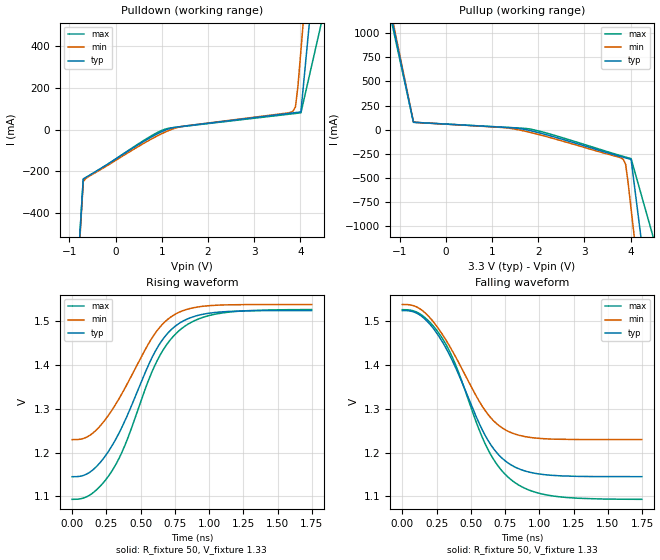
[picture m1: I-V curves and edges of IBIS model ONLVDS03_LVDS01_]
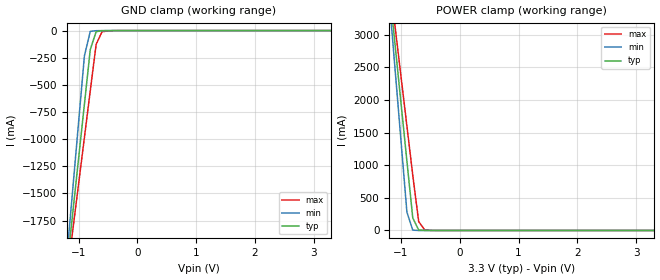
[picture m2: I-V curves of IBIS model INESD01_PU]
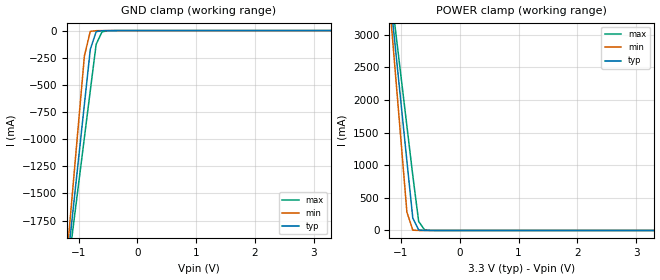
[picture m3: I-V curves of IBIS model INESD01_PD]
|   This file is an IBIS representation of the   |
|   Integrated Device Technology, Inc.   |
|   ICS844008I-01   |
|   FEMTOCLOCKS CRYSTAL-TO-LVDS FREQUENCY SYNTHESIZER   |
[IBIS Ver]   4.1
[File name]   844008i_01_3v3.ibs
[File Rev]   4.0
[Date]   15 Jul 2009 | Last modified
|   Mar 27 2006 | Generated
[Source]   Originated at Integrated Device Technology, Inc.
[Disclaimer]
IDT hereby grants the user of this IBIS model a non-exclusive,
nontransferable license to use this IBIS model under the following terms.
Before using this IBIS model, the user should read this license.
If the user does not accept these terms,  the IBIS model should be
returned to IDT within 30 days.
   The user is granted this license only to use the IBIS model and
is not granted rights to sell, load, rent, lease or license the IBIS
model in whole or in part, or in modified form to anyone other than
user. User may modify the IBIS model to suit its specific
applications but rights to derivative works and such modifications
shall belong to IDT.
   This IBIS model is provided on an "AS IS" basis and IDT makes
absolutely no warranty with respect to the information contained
herein. IDT DISCLAIMS AND CUSTOMER WAIVES ALL WARRANTIES, EXPRESS
OR IMPLIED, INCLUDING WARRANTIES OF MERCHANTABILITY OR FITNESS FOR
A PARTICULAR PURPOSE. The entire risk as to quality and performance
is with the Customer. ACCORDINGLY, IN NO EVENT SHALL THE COMPANY BE
LIABLE FOR ANY DAMAGES, WHETHER IN CONTRACT OR TORT,INCLUDING ANY
LOST PROFITS OR OTHER INCIDENTAL, CONSEQUENTIAL, EXEMPLARY, OR
PUNITIVE DAMAGES ARISING OUT OF THE USE OR APPLICATION OF THE IBIS
model provided in this package. Further, IDT reserves the right to
make changes without notice to any product herein to improve
reliability, function, or design. IDT does not convey any license
under patent rights or any other intellectual property rights,
including those of third parties.
   IDT is not obligated to provide maintenance or support
for the licensed IBIS model.
[Copyright]   Copyright 2008 by Integrated Device Technology, Inc.
[Component]   ICS844008YI-01
[Manufacturer] Integrated Device Technology, Inc.
[Package]
|LQFP32
|lead + wire   typ   min   max
R_pkg   220.4m   212.5m   238m
L_pkg   1.841n   1.708n   1.974n
C_pkg   0.316p   0.2907p   0.33p
[Pin] signal_name   model_name   R_pin   L_pin   C_pin
1   QA0   ONLVDS03_LVDS01_   238m   1.974n   0.330p
2   nQA0   ONLVDS03_LVDS01_   225m   1.841n   0.311p
3   VDD   POWER   218m   1.7745n   0.301p
4   QA1   ONLVDS03_LVDS01_   213m   1.708n   0.291p
5   nQA1   ONLVDS03_LVDS01_   213m   1.708n   0.291p
6   GND   GND   218m   1.7745n   0.301p
7   QA2   ONLVDS03_LVDS01_   225m   1.841n   0.311p
8   nQA2   ONLVDS03_LVDS01_   238m   1.974n   0.330p
9   F_SEL   INESD01_PU   238m   1.974n   0.330p
10   QA3   ONLVDS03_LVDS01_   225m   1.841n   0.311p
11   nQA3   ONLVDS03_LVDS01_   218m   1.7745n   0.301p
12   VDD   POWER   213m   1.708n   0.291p
13   GND   GND   213m   1.708n   0.291p
14   QB0   ONLVDS03_LVDS01_   218m   1.7745n   0.301p
15   nQB0   ONLVDS03_LVDS01_   225m   1.841n   0.311p
16   MR   INESD01_PD   238m   1.974n   0.330p
17   nQB1   ONLVDS03_LVDS01_   238m   1.974n   0.330p
18   QB1   ONLVDS03_LVDS01_   225m   1.841n   0.311p
19   GND   GND   218m   1.7745n   0.301p
20   nQB2   ONLVDS03_LVDS01_   213m   1.708n   0.291p
21   QB2   ONLVDS03_LVDS01_   213m   1.708n   0.291p
22   VDD   POWER   218m   1.7745n   0.301p
23   nQB3   ONLVDS03_LVDS01_   225m   1.841n   0.311p
24   QB3   ONLVDS03_LVDS01_   238m   1.974n   0.330p
25   VDDA   POWER   238m   1.974n   0.330p
26   nPLL_SEL   INESD01_PD   225m   1.841n   0.311p
27   VDD   POWER   218m   1.7745n   0.301p
28   OEB   INESD01_PU   213m   1.708n   0.291p
29   GND   GND   213m   1.708n   0.291p
30   XTAL_OUT   nc   218m   1.7745n   0.301p
31   XTAL_IN   nc   225m   1.841n   0.311p
32   OEA   INESD01_PU   238m   1.974n   0.330p
[Diff Pin]  inv_pin  vdiff tdelay_typ tdelay_min  tdelay_max
|Outputs
1   2   NA   0  0  0
4   5   NA   0  0  0
7   8   NA   0  0  0
10   11   NA   0  0  0
14   15   NA   0  0  0
18   17   NA   0  0  0
21   20   NA   0  0  0
24   23   NA   0  0  0
[Component]   ICS844008KI-01
[Manufacturer] Integrated Device Technology, Inc.
[Package]
|LD QFN 32
|lead + wire   typ   min   max
R_pkg   72.4655m   58.886m   86.045m
L_pkg   1.47175nH   1.11650nH   1.77850nH
C_pkg   0.07747pF   0.07444pF   0.08050pF
[Pin] signal_name   model_name   R_pin   L_pin   C_pin
1   QA0   ONLVDS03_LVDS01_   86.045m   1.77850nH   0.08050pF
2   nQA0   ONLVDS03_LVDS01_   76.996m   1.55783nH   0.07848pF
3   VDD   POWER   67.941m   1.33717nH   0.07646pF
4   QA1   ONLVDS03_LVDS01_   58.886m   1.11650nH   0.07444pF
5   nQA1   ONLVDS03_LVDS01_   58.886m   1.11650nH   0.07444pF
6   GND   GND   67.941m   1.33717nH   0.07646pF
7   QA2   ONLVDS03_LVDS01_   76.996m   1.55783nH   0.07848pF
8   nQA2   ONLVDS03_LVDS01_   86.045m   1.77850nH   0.08050pF
9   F_SEL   INESD01_PU   86.045m   1.77850nH   0.08050pF
10   QA3   ONLVDS03_LVDS01_   76.996m   1.55783nH   0.07848pF
11   nQA3   ONLVDS03_LVDS01_   67.941m   1.33717nH   0.07646pF
12   VDD   POWER   58.886m   1.11650nH   0.07444pF
13   GND   GND   58.886m   1.11650nH   0.07444pF
14   QB0   ONLVDS03_LVDS01_   67.941m   1.33717nH   0.07646pF
15   nQB0   ONLVDS03_LVDS01_   76.996m   1.55783nH   0.07848pF
16   MR   INESD01_PD   86.045m   1.77850nH   0.08050pF
17   nQB1   ONLVDS03_LVDS01_   86.045m   1.77850nH   0.08050pF
18   QB1   ONLVDS03_LVDS01_   76.996m   1.55783nH   0.07848pF
19   GND   GND   67.941m   1.33717nH   0.07646pF
20   nQB2   ONLVDS03_LVDS01_   58.886m   1.11650nH   0.07444pF
21   QB2   ONLVDS03_LVDS01_   58.886m   1.11650nH   0.07444pF
22   VDD   POWER   67.941m   1.33717nH   0.07646pF
23   nQB3   ONLVDS03_LVDS01_   76.996m   1.55783nH   0.07848pF
24   QB3   ONLVDS03_LVDS01_   86.045m   1.77850nH   0.08050pF
25   VDDA   POWER   86.045m   1.77850nH   0.08050pF
26   nPLL_SEL   INESD01_PD   76.996m   1.55783nH   0.07848pF
27   VDD   POWER   67.941m   1.33717nH   0.07646pF
28   OEB   INESD01_PU   58.886m   1.11650nH   0.07444pF
29   GND   GND   58.886m   1.11650nH   0.07444pF
30   XTAL_OUT   nc   67.941m   1.33717nH   0.07646pF
31   XTAL_IN   nc   76.996m   1.55783nH   0.07848pF
32   OEA   INESD01_PU   86.045m   1.77850nH   0.08050pF
[Diff Pin]  inv_pin  vdiff tdelay_typ tdelay_min  tdelay_max
|Outputs
1   2   NA   0  0  0
4   5   NA   0  0  0
7   8   NA   0  0  0
10   11   NA   0  0  0
14   15   NA   0  0  0
18   17   NA   0  0  0
21   20   NA   0  0  0
24   23   NA   0  0  0
| Models and submodels in the file (3): ONLVDS03_LVDS01_ (Output), INESD01_PU (Input), INESD01_PD (Input)
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[Model]   ONLVDS03_LVDS01_
Model_type   Output
Polarity   Non-Inverting
|   typ   min   max
C_comp   2pF   1.5pF   2.5pF
Vmeas = 1.33V
Rref = 50
Cref = 0
Vref = 1.33V
|   typ   min   max
[Voltage range]   3.3V   3.135V   3.465V
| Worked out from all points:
|   slope of the pulldown table from 0 to 0.495 V, typ, clamps not added: 7.11 ohm
|   slope of the pullup table from 0 to 0.495 V, typ, clamps not added: 37.1 ohm
|   rising waveform, R_fixture 50, V_fixture 1.33: 20-80 % time 339ps typ, 337ps min, 345ps max; typ from 1.15 V to 1.52 V
|   falling waveform, R_fixture 50, V_fixture 1.33: 20-80 % time 339ps typ, 337ps min, 345ps max; typ from 1.52 V to 1.15 V
[Pulldown]
|Voltage   I (typ)   I (min)   I (max)
-3.3V     -12.67A    -10.97A    -15.57A
-1.22V    -2.155A    -2.213A    -2.102A
-700mV    -236.2mA   -248.3mA   -238.7mA
-591mV    -221.6mA   -225.9mA   -223.9mA
921.3mV   -17.61mA   -27.52mA   -11.29mA
1.407V    15.22mA    14.4mA     14.35mA
3.838V    80.8mA     88.77mA    76.77mA
3.892V    82.3mA     109.8mA    78.15mA
3.946V    83.87mA    209.4mA    79.54mA
4.01V     86.01mA    380.6mA    81.18mA
4.528V    1.295A     1.771A     585.9mA
6.6V      7.985A     7.361A     9.102A
[Pullup]
|Voltage   I (typ)   I (min)   I (max)
-3.3V     7.977A     6.909A     9.772A
-1.22V    1.262A     1.3A       1.22A
-700mV    78.05mA    82.13mA    76.54mA
1.245V    25.16mA    22.28mA    26.55mA
1.786V    -4.761mA   -23mA      9.927mA
3.784V    -277.4mA   -290.3mA   -268.2mA
3.838V    -284.5mA   -305.2mA   -275.7mA
3.892V    -291.6mA   -357.9mA   -283.1mA
3.946V    -298.7mA   -552mA     -290.5mA
4.01V     -307.4mA   -820.6mA   -299.1mA
4.528V    -2.265A    -2.995A    -1.179A
6.6V      -12.7A     -11.71A    -14.49A
[Ramp]
|   typ   min   max
dV/dt_r   0.303/0.524n   0.247/0.507n   0.346/0.557n
dV/dt_f   0.303/0.524n   0.247/0.507n   0.346/0.557n
R_load =   50.0000
[Rising Waveform]
R_fixture = 50
V_fixture = 1.33   |Vcc_typ
V_fixture_min = 1.36 |Vcc_min
V_fixture_max = 1.33 |Vcc_max
C_fixture = 0.0p
| Time   typ   min   max
0s        1.145V     1.229V     1.093V
141.9ps   1.158V     1.242V     1.106V
289ps     1.214V     1.296V     1.157V
388.9ps   1.275V     1.349V     1.219V
613.1ps   1.435V     1.476V     1.405V
700.7ps   1.474V     1.505V     1.451V
798.8ps   1.498V     1.523V     1.483V
924.9ps   1.514V     1.533V     1.506V
1.093ns   1.521V     1.537V     1.519V
1.748ns   1.524V     1.538V     1.527V
[Falling Waveform]
R_fixture = 50
V_fixture = 1.33   |Vcc_typ
V_fixture_min = 1.36 |Vcc_min
V_fixture_max = 1.33 |Vcc_max
C_fixture = 0.0p
| Time   typ   min   max
0s        1.525V     1.539V     1.527V
141.9ps   1.512V     1.526V     1.515V
289ps     1.455V     1.472V     1.463V
388.9ps   1.395V     1.419V     1.401V
613.1ps   1.235V     1.293V     1.215V
700.7ps   1.196V     1.263V     1.169V
798.8ps   1.171V     1.245V     1.137V
924.9ps   1.156V     1.235V     1.115V
1.093ns   1.148V     1.231V     1.101V
1.748ns   1.145V     1.23V      1.093V
[Model]   INESD01_PU
Model_type   Input
Polarity   Non-Inverting
Vinl = 0.8V
Vinh = 2.0V
|   typ   min   max
C_comp   2pF   1.5pF   2.5pF
|   typ   min   max
[Voltage range]  3.3V   3.15V   3.45V
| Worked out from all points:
|   GND clamp passes 1 mA (typ) near -0.55 V on its own axis
|   POWER clamp passes 1 mA (typ) near -0.61 V on its own axis
[GND_clamp]
|Voltage   I(typ)   I(min)   I(max)
-3.3V     -12.83A    -15.14A    -11.37A
-1.2V     -2.195A    -2.092A    -2.281A
-1.1V     -1.689A    -1.472A    -1.849A
-900mV    -678.5mA   -232.7mA   -984.8mA
-800mV    -174mA     -7.237mA   -553.3mA
-700mV    -9.767mA   -1.114mA   -126.1mA
-600mV    -1.7mA     -240.1uA   -11.15mA
-300mV    -81.66uA   -67.79uA   -163.4uA
3.3V      1.866nA    1.113pA    239.1nA
[POWER_clamp]
|Voltage   I(typ)   I(min)   I(max)
-3.3V     22.38A     26.45A     19.82A
-1.2V     3.723A     3.545A     3.874A
-1.1V     2.836A     2.457A     3.116A
-1V       1.949A     1.369A     2.358A
-900mV    1.063A     281mA      1.601A
-800mV    191.5mA    5.012mA    843.9mA
-700mV    8.032mA    142.2uA    138.3mA
-600mV    607uA      17.63uA    10.62mA
-400mV    16.32uA    7.545uA    335.9uA
3.3V      -71.13uA   -62.11uA   -78.26uA
[Model]   INESD01_PD
Model_type   Input
Polarity   Non-Inverting
Vinl = 0.80V
Vinh = 2.0V
|   typ   min   max
C_comp   2pF   1.5pF   2.5pF
|   typ   min   max
[Voltage range]  3.3V   3.15V   3.45V
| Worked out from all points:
|   GND clamp passes 1 mA (typ) near -0.55 V on its own axis
|   POWER clamp passes 1 mA (typ) near -0.60 V on its own axis
[GND_clamp]
|Voltage I(typ)   I(min)   I(max)
-3.3V     -12.83A    -15.14A    -11.37A
-1.2V     -2.195A    -2.092A    -2.281A
-1.1V     -1.689A    -1.472A    -1.849A
-900mV    -678.5mA   -232.6mA   -984.8mA
-800mV    -173.9mA   -7.175mA   -553.2mA
-700mV    -9.696mA   -1.052mA   -126mA
-600mV    -1.629mA   -178uA     -11.07mA
-300mV    -10.53uA   -5.678uA   -86.08uA
3.3V      71.13uA    62.11uA    77.58uA
[POWER_clamp]
|Voltage   I(typ)   I(min)   I(max)
-3.3V     22.38A     26.45A     19.82A
-1.2V     3.723A     3.545A     3.874A
-1.1V     2.836A     2.457A     3.116A
-1V       1.949A     1.369A     2.358A
-900mV    1.063A     281.1mA    1.601A
-800mV    191.6mA    5.074mA    844mA
-700mV    8.104mA    204.3uA    138.4mA
-600mV    678.1uA    79.74uA    10.7mA
-400mV    87.44uA    69.65uA    413.2uA
3.3V      -3.041nA   -425fA     -919.9nA
